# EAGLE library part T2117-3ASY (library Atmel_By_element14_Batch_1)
Zero-Voltage Switch with Adjustable Ramp
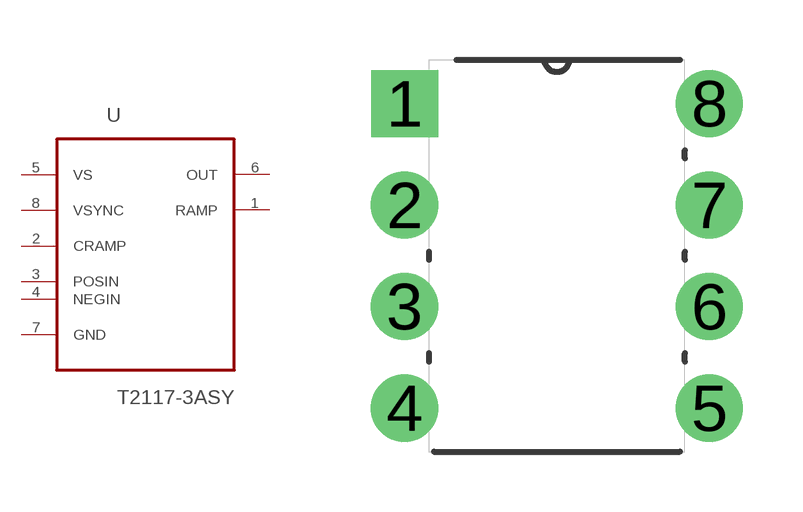
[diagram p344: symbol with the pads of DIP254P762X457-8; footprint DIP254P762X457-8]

Designator prefix U

## T2117-3ASY (MPN: T2117-3ASY; OC_FARNELL: 1455171; OC_NEWARK: 59M3051; PACKAGE: PDIP-8; SUPPLIER: Atmel)  [DIP254P762X457-8]
1  RAMP  out
2  CRAMP  pas
3  POSIN  in
4  NEGIN  in
5  VS  pwr
6  OUT  out
7  GND  pas
8  VSYNC  in

## Footprint DIP254P762X457-8 (pad centres in mm)
drill 1.118 square: 1 -7.62,7.62
drill 1.118: 2 -7.62,5.08; 3 -7.62,2.54; 4 -7.62,0; 5 0,0; 6 0,2.54; 7 0,5.08; 8 0,7.62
